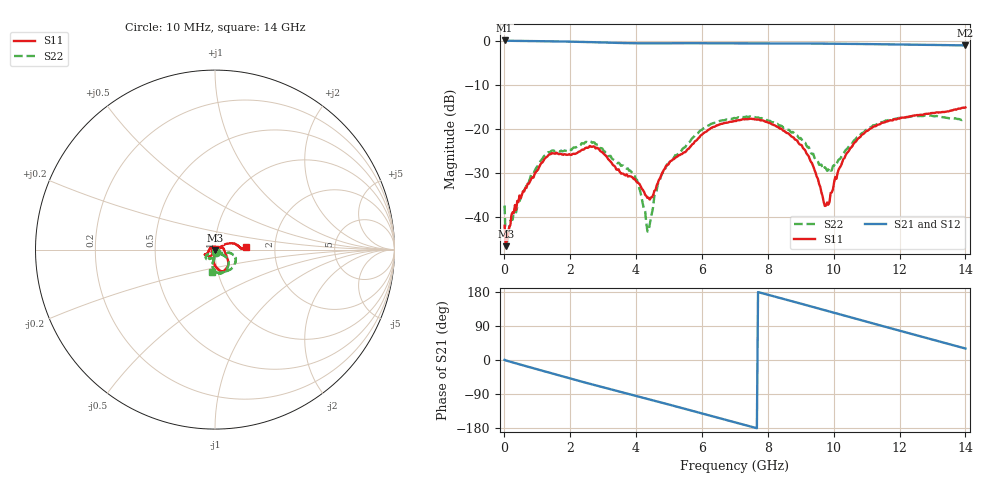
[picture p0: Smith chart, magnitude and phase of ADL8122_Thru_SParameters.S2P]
! "Analog Devices, Inc."
! Device:	ADL8122ACPZN - THRU
! Description:	"10 kHz to 10 GHz, Wideband, Low Noise Amplifier"
! Conditions:	Pin = -25 dBm
!		Operating Temperature = +25 C (at package bottom)
! Measurement used thru-cal line of SN#1.
! Frequency (GHz)	S11_Mag (dB)	S11_Phase (deg)	S21_Mag (dB)	S21_Phase (deg)	S12_Mag (dB)	S12_Phase (deg)	S22_Mag (dB)	S22_Phase (deg)
#  GHZ  S  DB  R 50
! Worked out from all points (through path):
!   401 points, 10 MHz to 14 GHz, reference 50 ohm
!   highest |S21| = 0.05 dB at 10 MHz (marker M1); lowest = -1.1 dB at 14 GHz (marker M2)
!   group delay of S21, straight-line fit = 65.1 ps
!   lowest |S11| = -46.7 dB at 44.98 MHz (marker M3), VSWR 1.01, Z = 50 - j0.46 ohm
!   |S11| at or under -10 dB: start of sweep to end of sweep
!   |S22| runs from -46.4 to -17.0 dB; largest |S21 - S12| = 0.0065
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0.01  -42.08 -81.5  0.05 0.4  -0.00 0.4  -37.49 -67.0
0.044975  -46.74 -90.3  -0.01 -1.1  -0.01 -1.1  -46.38 -87.0
0.114925  -44.15 -81.0  -0.01 -3.0  -0.01 -2.9  -44.75 -125.8
0.394725  -36.47 -79.5  -0.05 -9.8  -0.05 -9.8  -37.77 -105.9
1.2691  -26.52 -123.9  -0.12 -31.0  -0.12 -31.0  -25.84 -105.5
2.353325  -24.82 -153.1  -0.27 -57.1  -0.27 -57.1  -23.31 -123.7
2.808  -24.36 -152.2  -0.37 -67.9  -0.37 -67.9  -23.62 -141.3
3.892225  -31.09 152.2  -0.58 -92.6  -0.57 -92.6  -30.08 -139.7
4.0671  -32.30 143.8  -0.59 -96.5  -0.59 -96.5  -32.86 -140.8
4.381875  -35.71 94.5  -0.60 -103.5  -0.60 -103.5  -43.36 -86.0
4.69665  -31.63 34.2  -0.60 -110.7  -0.59 -110.6  -32.10 -31.5
5.011425  -27.73 17.1  -0.59 -117.8  -0.59 -117.8  -27.68 -35.4
5.8858  -22.23 -31.9  -0.57 -138.3  -0.57 -138.3  -20.99 -37.9
7.005  -18.25 -59.3  -0.61 -164.5  -0.61 -164.5  -17.61 -65.3
8.369025  -19.98 -84.6  -0.65 163.7  -0.65 163.7  -19.37 -95.6
9.348325  -27.93 -95.8  -0.65 140.6  -0.66 140.5  -25.79 -97.2
9.803  -36.80 -24.1  -0.67 129.7  -0.67 129.7  -29.62 -58.2
10.2227  -28.44 26.1  -0.70 119.6  -0.69 119.6  -26.57 -22.2
10.57245  -23.93 27.4  -0.72 111.2  -0.72 111.3  -23.18 -13.8
11.69165  -18.17 12.6  -0.84 84.7  -0.84 84.7  -17.90 -23.5
12.77587  -16.67 2.5  -0.94 59.2  -0.94 59.1  -17.02 -48.1
14  -15.17 4.7  -1.07 30.3  -1.07 30.3  -18.17 -96.9
